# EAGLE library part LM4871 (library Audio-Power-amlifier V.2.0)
The LM4871 is a mono bridged audio power amplifier capable of delivering 3W of continuous average power into a 3Ω load with less than 10% THD when powered by a 5V power supply (see Note). To conserve power in portable applications, the LM4871's micropower shutdown mode (IQ = 0.6μA, typ) is activated when VDD is applied to the SHUTDOWN pin. Boomer audio power amplifiers are designed specifically to provide high power, high fidelity audio output. They require few external components and operate on low supply voltages from 2.0V to 5.5V. Since the LM4871 does not require output coupling capacitors, bootstrap capacitors, or snubber networks, it is ideally suited for lowpower portable systems that require minimum volume and weight.
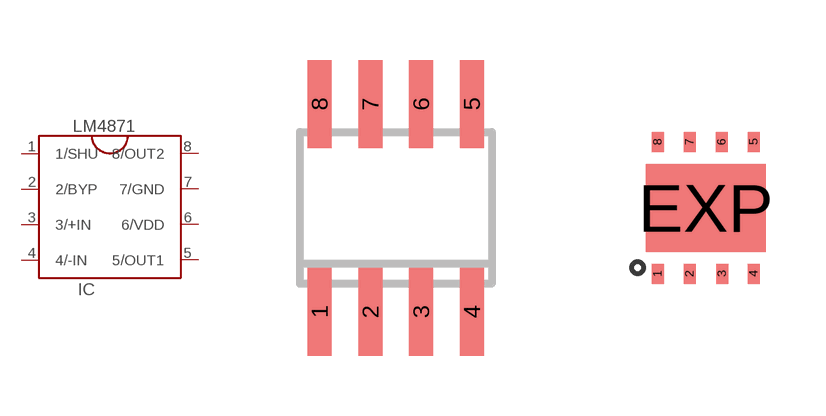
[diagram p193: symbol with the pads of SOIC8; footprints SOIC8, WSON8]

Designator prefix IC

## LM4871LM4871MX/NOPB  [SOIC8]
1  1/SHU
2  2/BYP
3  3/+IN  in
4  4/-IN  in
5  5/OUT1  out
6  6/VDD  pwr
7  7/GND  pwr
8  8/OUT2  out

## LM4871LM4871LDX/NOPB  [WSON8]
Pads as for SOIC8

## LM4871LM4871MMX/NOPB  [VSSOP8]
Pads as for SOIC8

## Footprint SOIC8 (pad centres in mm)
Small Outline IC
smd 0.6 x 2.2: 1 -1.905,-2.6; 2 -0.635,-2.6; 3 0.635,-2.6; 4 1.905,-2.6; 5 1.905,2.6; 6 0.635,2.6; 7 -0.635,2.6; 8 -1.905,2.6

## Footprint WSON8 (pad centres in mm)
LLP4x4 body. http://www.ti.com/sc/docs/package/guide.htm
smd 0.3 x 0.5: 1 -1.2,-1.65; 2 -0.4,-1.65; 3 0.41,-1.65; 4 1.2,-1.65; 5 1.2,1.65; 6 0.4,1.65; 7 -0.4,1.65; 8 -1.2,1.65
smd 3 x 2.2: EXP 0,0

## Footprint VSSOP8 (pad centres in mm)
LGA 4x4 DGK. www.ti.com/audio
smd 0.305 x 0.61: 1 -1.2,-1.65; 2 -0.4,-1.65; 3 0.4,-1.65; 4 1.2,-1.65; 5 1.2,1.65; 6 0.4,1.65; 7 -0.4,1.65; 8 -1.2,1.65
smd 3 x 2.2: EXP 0,0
